TYPE series5x_PDin :
STRUCT
	Caneoseries5x_TouchZone1 AT %I* : USINT;
	Caneoseries5x_TouchZone2 AT %I* : USINT;
	Caneoseries5x_TouchZone3 AT %I* : USINT;
	Caneoseies5x_TouchZone4 AT %I* : USINT;
END_STRUCT
END_TYPE
